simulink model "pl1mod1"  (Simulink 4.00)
settings: Solver=ode45  StartTime=0.0  StopTime=5  RelTol=1e-3

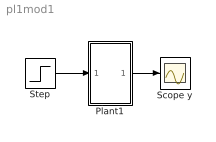
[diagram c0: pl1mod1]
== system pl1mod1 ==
  Plant1 : Subsystem
  Scope y : Scope
  Step : Step  Time=0  Before=0  After=1  SampleTime=0
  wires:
  Step/1 -> Plant1/1(u)
  Plant1/1(y) -> Scope y/1

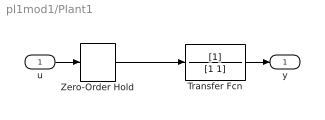
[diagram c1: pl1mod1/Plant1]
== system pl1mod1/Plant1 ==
  u : Inport  Port=1  LatchInput=off
  Transfer Fcn : TransferFcn  Numerator=[1]  Denominator=[1 1]  AbsoluteTolerance=auto  Realization=auto
  Zero-Order Hold : ZeroOrderHold  SampleTime=0.1
  y : Outport  Port=1
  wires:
  Zero-Order Hold/1 -> Transfer Fcn/1
  u/1 -> Zero-Order Hold/1
  Transfer Fcn/1 -> y/1
